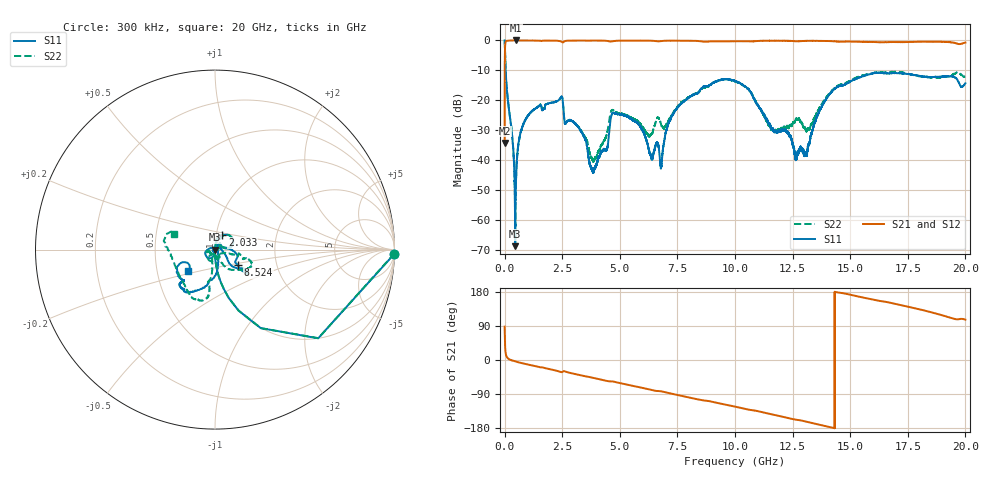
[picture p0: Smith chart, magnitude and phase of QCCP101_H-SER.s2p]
!{QCCP101}
!Johanson Technology Inc.
!www.johansontechnology.com
!Test Board Conditions:
!Substrate Type  RO4350B
!Substrate Thickness  20 mil
!Substrate Dk  3.66
!TL Type: GCPW
!TL Trace Width  36 mil
!TL Gap  12 mil
!Electrode orientation  Horizontal
!DUT TOPOLOGY	SERIES
!Mounting Pad LxW  26x36 mil
! Created Sat Jan  9 18:32:46 2021
# hz S ma R 50
! 2 Port Network Data from SP1.SP block
! freq  magS11  angS11  magS21  angS21  magS12  angS12  magS22  angS22
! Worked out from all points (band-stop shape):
!   20001 points, 300 kHz to 20 GHz, reference 50 ohm
!   highest |S21| = 0.00 dB at 478.3 MHz (marker M1); lowest = -34.3 dB at 300 kHz (marker M2)
!   |S21| within 3 dB of the highest: 15.63 MHz to end of sweep
!   lowest |S11| = -68.8 dB at 461.3 MHz (marker M3), VSWR 1.00, Z = 50 + j0.00447 ohm
!   |S11| at or under -10 dB: 46.01 MHz to end of sweep
!   |S22| runs from -62.0 to 0.0 dB; largest |S21 - S12| = 0.016
!   S11 on the Smith chart (normalised r, x): 300 kHz: 1, -83; 2.033 GHz: 1.07, +0.17; 8.524 GHz: 1.27, -0.23; 20 GHz: 0.72, -0.18
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300000  0.9996 -1.4  0.01937 88.0  0.01955 88.6  0.9986 -1.3
1.073e8  0.1366 -83.0  0.9895 6.9  0.9897 6.8  0.1368 -82.9
4.613e8  0.0003624 172.9  0.9998 -3.8  0.9988 -3.8  0.001242 -24.7
4.783e8  0.002494 98.1  1 -4.1  0.9986 -4.1  0.002394 68.2
8.893e8  0.04603 81.3  0.9976 -10.2  0.9978 -10.2  0.04568 77.2
2.0333e9  0.09064 63.5  0.9934 -25.2  0.9933 -25.2  0.09113 65.3
3.3343e9  0.0296 56.1  0.9959 -40.7  0.9953 -40.7  0.03047 39.6
3.8333e9  0.006295 119.9  0.9952 -47.0  0.9957 -47.0  0.009808 -34.3
4.4193e9  0.01497 -137.4  0.985 -55.1  0.9861 -55.2  0.02581 -88.4
4.7443e9  0.06068 -143.2  0.98 -57.3  0.9792 -57.2  0.06663 -122.8
5.7893e9  0.04051 179.8  0.992 -71.1  0.9922 -71.1  0.04474 -131.4
6.2623e9  0.01497 130.9  0.9912 -77.4  0.9909 -77.4  0.02521 -93.0
6.6673e9  0.01821 -39.8  0.9664 -82.0  0.9658 -81.9  0.05036 -65.4
7.4453e9  0.06971 6.3  0.9913 -91.5  0.9907 -91.5  0.07313 -15.6
8.5243e9  0.1557 -33.8  0.9686 -105.6  0.9677 -105.6  0.1533 -12.3
1.00003e10  0.2096 -37.2  0.9704 -123.0  0.9695 -123.0  0.2049 -31.3
1.16363e10  0.03415 7.3  0.9879 -143.9  0.9892 -144.0  0.0326 -114.8
1.26583e10  0.01075 67.0  0.9698 -157.6  0.9718 -157.7  0.0491 -162.3
1.33343e10  0.02885 -52.0  0.9851 -166.2  0.9873 -166.2  0.04025 -118.7
1.43803e10  0.1608 -93.4  0.964 179.3  0.9667 179.3  0.1672 -99.3
1.66673e10  0.281 -129.0  0.9372 151.9  0.9328 151.6  0.296 -110.3
2e10  0.1923 -140.7  0.9211 106.5  0.9155 106.3  0.2465 159.6
